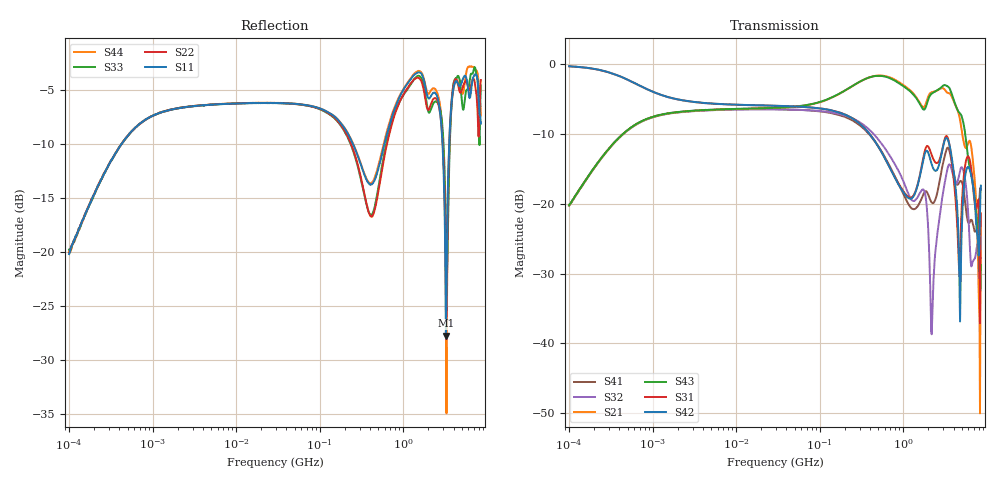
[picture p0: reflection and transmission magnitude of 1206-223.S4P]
!Agilent Technologies,E5071C,MY46110495,A.10.06
!Date: Tue Jun 06 12:56:32 2017
!Data & Calibration Information:
!Freq	S11:SOLT4(ON)	S12:SOLT4(ON)	S13:SOLT4(ON)	S14:SOLT4(ON)
!	S21:SOLT4(ON)	S22:SOLT4(ON)	S23:SOLT4(ON)	S24:SOLT4(ON)
!	S31:SOLT4(ON)	S32:SOLT4(ON)	S33:SOLT4(ON)	S34:SOLT4(ON)
!	S41:SOLT4(ON)	S42:SOLT4(ON)	S43:SOLT4(ON)	S44:SOLT4(ON)
!PortZ  Port1:50+j0  Port2:50+j0  Port3:50+j0  Port4:50+j0
!Above PortZ is port z conversion or system Z0 setting when saving the data.
!When reading, reference impedance value at option line is always used.
# Hz S dB R 50
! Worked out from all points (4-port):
!   801 points, 100 kHz to 8.5 GHz, reference 50 ohm
!   strongest paths, dB at 100 kHz, 1.721 MHz, 29.51 MHz, 502.3 MHz, 8.5 GHz:
!     S42: -0.3, -4.8, -5.9, -11.8, -17.4
!     S31: -0.3, -4.9, -5.9, -11.8, -21.4
!     S43: -20.2, -6.9, -6.2, -1.6, -28.8
!     S21: -20.2, -7.0, -6.2, -1.6, -26.8
!     S32: -20.3, -7.0, -6.4, -10.8, -27.8
!     S41: -20.3, -7.0, -6.4, -11.8, -18.0
!   lowest |S11| = -27.7 dB at 3.239 GHz (marker M1), VSWR 1.09, Z = 54.3 - j0.00434 ohm
!   |S11| at or under -10 dB: start of sweep to 427 kHz; 249.6 MHz to 595.1 MHz (345.5 MHz wide, 81.8 % of centre); 2.95 GHz to 3.549 GHz (599.7 MHz wide, 18.5 % of centre)
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100000  -20.19 72.3  -20.21 77.1  -0.27 -5.4  -20.28 -103.1
        -20.23 76.9  -20.08 70.9  -20.27 -103.1  -0.28 -5.4
        -0.28 -5.5  -20.25 -103.4  -19.78 74.1  -20.24 76.3
        -20.27 -102.9  -0.25 -5.5  -20.22 76.8  -19.94 72.3
1.858222e8  -8.28 -11.8  -4.00 15.1  -7.02 -44.8  -7.41 136.4
            -4.01 15.1  -8.46 -17.3  -7.22 131.3  -7.06 -44.7
            -7.03 -44.7  -7.23 131.3  -8.53 -17.6  -3.99 14.9
            -7.39 136.4  -7.04 -44.7  -3.98 14.9  -8.23 -12.0
2.219465e9  -5.41 71.3  -3.95 -9.3  -13.17 69.1  -19.88 -165.0
            -3.96 -9.3  -6.09 80.5  -36.96 134.5  -14.55 68.9
            -13.17 69.2  -36.65 132.2  -6.55 80.3  -4.16 -6.5
            -19.86 -164.8  -14.53 69.0  -4.14 -6.5  -4.95 71.2
3.239055e9  -27.73 -0.1  -3.84 -28.2  -10.31 32.3  -12.52 78.9
            -3.85 -28.2  -21.88 109.4  -16.09 46.6  -10.57 35.7
            -10.31 32.5  -16.10 46.7  -17.88 113.2  -3.03 -25.8
            -12.50 79.3  -10.59 35.8  -3.01 -25.8  -24.75 77.8
5.311123e9  -3.83 -75.2  -11.18 -54.4  -15.98 54.3  -18.22 -70.5
            -11.21 -54.2  -4.47 -75.4  -15.51 -60.9  -17.70 62.7
            -15.99 54.3  -15.52 -60.8  -6.68 -80.6  -8.70 -66.5
            -18.24 -70.4  -17.70 62.8  -8.70 -66.4  -5.00 -64.5
6.738951e9  -4.17 15.8  -13.24 -71.9  -16.61 -19.5  -22.64 79.7
            -13.22 -71.9  -4.06 9.2  -28.40 65.8  -16.94 -6.2
            -16.62 -19.2  -28.38 65.8  -3.53 12.0  -16.65 -71.0
            -22.62 79.9  -16.93 -5.8  -16.62 -70.9  -2.90 7.6
8.5e9  -8.15 111.0  -26.78 87.9  -21.35 54.0  -18.01 24.4
       -26.77 88.2  -4.12 125.9  -27.76 23.0  -17.42 36.6
       -21.37 54.4  -27.78 23.5  -4.61 125.3  -28.91 111.3
       -18.00 24.8  -17.39 37.0  -28.77 111.6  -7.38 97.1
